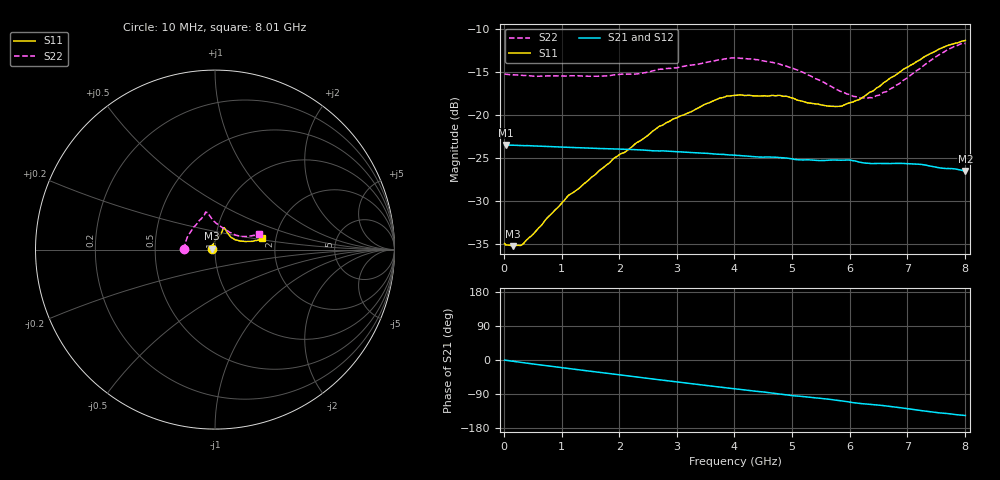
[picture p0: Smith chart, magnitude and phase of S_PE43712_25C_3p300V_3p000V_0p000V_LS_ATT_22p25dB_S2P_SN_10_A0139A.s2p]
! DEVICE ID: PE43712
! File Path: z:\PE43713\PE43713_CHAR_NOM_04292014\AMB\3p300\LS_ATT_22p25dB\PE43713_AMB_3p300V_3p000V_0p000V_LS_ATT_22p25dB_S2P_SN_10_A0139A.s2p
! Serial: 10
! Lot: A0139A
! Temp: 25C
! VDD: 3.300
! VSS: 0.000
! Control_Hi: 3.000
! Control_Lo: 0.000
! Attenuation Step: 22.25dB
! Port 1: RF1
! Port 2: RF2
! ThroughPath:1-2
! IDD: 0.0001470566
! ISS: -7.97e-008
#  Hz  S  RI  R  50
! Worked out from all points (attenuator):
!   801 points, 10 MHz to 8.01 GHz, reference 50 ohm
!   highest |S21| = -23.50 dB at 30 MHz (marker M1); lowest = -26.5 dB at 8.01 GHz (marker M2)
!   lowest |S11| = -35.3 dB at 160 MHz (marker M3), VSWR 1.04, Z = 48.4 + j0.523 ohm
!   |S11| at or under -10 dB: start of sweep to end of sweep
!   |S22| runs from -18.1 to -11.7 dB; largest |S21 - S12| = 0.00024
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1e7  -0.0179 0.000681  0.0669 -0.000326  0.0669 -0.000311  -0.173 0.00121
3e7  -0.0175 0.00167  0.0669 -0.000793  0.0669 -0.000802  -0.1724 0.00301
1.6e8  -0.0164 0.0054  0.0665 -0.00402  0.0666 -0.00401  -0.1708 0.0121
3.3e8  -0.0149 0.00967  0.0658 -0.0081  0.0658 -0.00802  -0.1684 0.0221
1.1e9  -0.00995 0.0321  0.0601 -0.0244  0.0601 -0.0244  -0.1536 0.0696
1.35e9  -0.00634 0.0383  0.0575 -0.0291  0.0575 -0.0291  -0.1467 0.0828
1.91e9  0.00515 0.0559  0.0505 -0.0385  0.0505 -0.0384  -0.1254 0.1165
2.34e9  0.0167 0.0681  0.044 -0.0447  0.044 -0.0447  -0.1055 0.138
2.68e9  0.0272 0.0808  0.0383 -0.0484  0.0383 -0.0484  -0.0885 0.1614
3.71e9  0.0448 0.1156  0.0195 -0.0558  0.0194 -0.0559  -0.0556 0.2006
4.01e9  0.0473 0.1213  0.0139 -0.0567  0.0139 -0.0567  -0.0523 0.2081
4.31e9  0.0477 0.1202  0.00853 -0.0567  0.00861 -0.0567  -0.0445 0.2067
4.75e9  0.054 0.1181  0.000808 -0.0567  0.000858 -0.0567  -0.0329 0.1966
5.35e9  0.0685 0.0943  -0.0087 -0.054  -0.00869 -0.054  -0.0146 0.1661
5.82e9  0.0875 0.0701  -0.0162 -0.0521  -0.0161 -0.0522  0.0199 0.1367
6.17e9  0.1094 0.0561  -0.0222 -0.0483  -0.0221 -0.0484  0.0549 0.1129
6.4e9  0.1277 0.0512  -0.0241 -0.0463  -0.024 -0.0463  0.0809 0.0966
6.68e9  0.155 0.0465  -0.0277 -0.0442  -0.0276 -0.0442  0.1139 0.0813
7.16e9  0.1988 0.046  -0.0345 -0.0387  -0.0344 -0.0387  0.1651 0.0735
7.55e9  0.2356 0.0518  -0.0375 -0.0321  -0.0373 -0.0322  0.2095 0.078
7.81e9  0.2536 0.0581  -0.039 -0.029  -0.039 -0.029  0.2351 0.0841
8.01e9  0.2637 0.0633  -0.0394 -0.0262  -0.0393 -0.0262  0.2468 0.085
